//{{V2}}
DATA_BLOCK DB2000

AUTHOR:WinCoCT
FAMILY:nb
NAME:0
VERSION:00.01


       STRUCT
         VAR0:STRUCT
            VAR1:WORD
            VAR2:BYTE
            VAR3:BYTE
            VAR4:DWORD
            VAR5:BYTE
            VAR6:BYTE
            VAR7:WORD
            VAR8:BYTE
            VAR9:WORD
            VAR10:BYTE
            VAR11:WORD
            VAR12:BYTE
            VAR13:WORD
            VAR14:BYTE
            VAR15:BYTE
            VAR16:BYTE
            VAR17:BYTE
            VAR18:BYTE
            VAR19:BYTE
            VAR20:BYTE
            VAR21:BYTE
            VAR22:WORD
            VAR23:WORD
         END_STRUCT
         VAR24:STRUCT
            VAR25:WORD
            VAR26:ARRAY [0..1735] of BYTE
         END_STRUCT
         VAR27:STRUCT
            VAR28:WORD
            VAR29:ARRAY [0..79] of BYTE
         END_STRUCT
       END_STRUCT
BEGIN

       VAR0.VAR1:=W#16#0024
       VAR0.VAR2:=B#16#00
       VAR0.VAR3:=B#16#01
       VAR0.VAR4:=DW#16#00000195
       VAR0.VAR5:=B#16#01
       VAR0.VAR6:=B#16#00
       VAR0.VAR7:=W#16#0010
       VAR0.VAR8:=B#16#10
       VAR0.VAR9:=W#16#0010
       VAR0.VAR10:=B#16#10
       VAR0.VAR11:=W#16#0080
       VAR0.VAR12:=B#16#50
       VAR0.VAR13:=W#16#0080
       VAR0.VAR14:=B#16#50
       VAR0.VAR15:=B#16#02
       VAR0.VAR16:=B#16#32
       VAR0.VAR17:=B#16#01
       VAR0.VAR18:=B#16#00
       VAR0.VAR19:=B#16#01
       VAR0.VAR20:=B#16#00
       VAR0.VAR21:=B#16#00
       VAR0.VAR22:=W#16#0100
       VAR0.VAR23:=W#16#26F5
       VAR24.VAR25:=W#16#06CA
       VAR24.VAR26[0]:=B#16#4D
       VAR24.VAR26[1]:=B#16#41
       VAR24.VAR26[2]:=B#16#0A
       VAR24.VAR26[3]:=B#16#06
       VAR24.VAR26[4]:=B#16#00
       VAR24.VAR26[5]:=B#16#00
       VAR24.VAR26[6]:=B#16#FE
       VAR24.VAR26[7]:=B#16#FF
       VAR24.VAR26[8]:=B#16#A2
       VAR24.VAR26[9]:=B#16#00
       VAR24.VAR26[10]:=B#16#00
       VAR24.VAR26[11]:=B#16#00
       VAR24.VAR26[12]:=B#16#80
       VAR24.VAR26[13]:=B#16#1F
       VAR24.VAR26[14]:=B#16#00
       VAR24.VAR26[15]:=B#16#04
       VAR24.VAR26[16]:=B#16#00
       VAR24.VAR26[17]:=B#16#00
       VAR24.VAR26[18]:=B#16#00
       VAR24.VAR26[19]:=B#16#03
       VAR24.VAR26[20]:=B#16#00
       VAR24.VAR26[21]:=B#16#00
       VAR24.VAR26[22]:=B#16#00
       VAR24.VAR26[23]:=B#16#81
       VAR24.VAR26[24]:=B#16#1F
       VAR24.VAR26[25]:=B#16#04
       VAR24.VAR26[26]:=B#16#04
       VAR24.VAR26[27]:=B#16#00
       VAR24.VAR26[28]:=B#16#00
       VAR24.VAR26[29]:=B#16#00
       VAR24.VAR26[30]:=B#16#07
       VAR24.VAR26[31]:=B#16#03
       VAR24.VAR26[32]:=B#16#F4
       VAR24.VAR26[33]:=B#16#01
       VAR24.VAR26[34]:=B#16#00
       VAR24.VAR26[35]:=B#16#14
       VAR24.VAR26[36]:=B#16#01
       VAR24.VAR26[37]:=B#16#04
       VAR24.VAR26[38]:=B#16#00
       VAR24.VAR26[39]:=B#16#00
       VAR24.VAR26[40]:=B#16#00
       VAR24.VAR26[41]:=B#16#01
       VAR24.VAR26[42]:=B#16#02
       VAR24.VAR26[43]:=B#16#00
       VAR24.VAR26[44]:=B#16#80
       VAR24.VAR26[45]:=B#16#00
       VAR24.VAR26[46]:=B#16#16
       VAR24.VAR26[47]:=B#16#00
       VAR24.VAR26[48]:=B#16#01
       VAR24.VAR26[49]:=B#16#00
       VAR24.VAR26[50]:=B#16#00
       VAR24.VAR26[51]:=B#16#00
       VAR24.VAR26[52]:=B#16#00
       VAR24.VAR26[53]:=B#16#01
       VAR24.VAR26[54]:=B#16#14
       VAR24.VAR26[55]:=B#16#01
       VAR24.VAR26[56]:=B#16#04
       VAR24.VAR26[57]:=B#16#00
       VAR24.VAR26[58]:=B#16#00
       VAR24.VAR26[59]:=B#16#00
       VAR24.VAR26[60]:=B#16#01
       VAR24.VAR26[61]:=B#16#03
       VAR24.VAR26[62]:=B#16#00
       VAR24.VAR26[63]:=B#16#80
       VAR24.VAR26[64]:=B#16#01
       VAR24.VAR26[65]:=B#16#16
       VAR24.VAR26[66]:=B#16#00
       VAR24.VAR26[67]:=B#16#01
       VAR24.VAR26[68]:=B#16#00
       VAR24.VAR26[69]:=B#16#00
       VAR24.VAR26[70]:=B#16#00
       VAR24.VAR26[71]:=B#16#00
       VAR24.VAR26[72]:=B#16#02
       VAR24.VAR26[73]:=B#16#14
       VAR24.VAR26[74]:=B#16#01
       VAR24.VAR26[75]:=B#16#04
       VAR24.VAR26[76]:=B#16#00
       VAR24.VAR26[77]:=B#16#00
       VAR24.VAR26[78]:=B#16#00
       VAR24.VAR26[79]:=B#16#01
       VAR24.VAR26[80]:=B#16#04
       VAR24.VAR26[81]:=B#16#00
       VAR24.VAR26[82]:=B#16#80
       VAR24.VAR26[83]:=B#16#02
       VAR24.VAR26[84]:=B#16#16
       VAR24.VAR26[85]:=B#16#00
       VAR24.VAR26[86]:=B#16#01
       VAR24.VAR26[87]:=B#16#00
       VAR24.VAR26[88]:=B#16#00
       VAR24.VAR26[89]:=B#16#00
       VAR24.VAR26[90]:=B#16#00
       VAR24.VAR26[91]:=B#16#03
       VAR24.VAR26[92]:=B#16#14
       VAR24.VAR26[93]:=B#16#01
       VAR24.VAR26[94]:=B#16#04
       VAR24.VAR26[95]:=B#16#00
       VAR24.VAR26[96]:=B#16#00
       VAR24.VAR26[97]:=B#16#00
       VAR24.VAR26[98]:=B#16#01
       VAR24.VAR26[99]:=B#16#05
       VAR24.VAR26[100]:=B#16#00
       VAR24.VAR26[101]:=B#16#80
       VAR24.VAR26[102]:=B#16#03
       VAR24.VAR26[103]:=B#16#16
       VAR24.VAR26[104]:=B#16#00
       VAR24.VAR26[105]:=B#16#01
       VAR24.VAR26[106]:=B#16#00
       VAR24.VAR26[107]:=B#16#00
       VAR24.VAR26[108]:=B#16#00
       VAR24.VAR26[109]:=B#16#00
       VAR24.VAR26[110]:=B#16#04
       VAR24.VAR26[111]:=B#16#14
       VAR24.VAR26[112]:=B#16#01
       VAR24.VAR26[113]:=B#16#04
       VAR24.VAR26[114]:=B#16#00
       VAR24.VAR26[115]:=B#16#00
       VAR24.VAR26[116]:=B#16#00
       VAR24.VAR26[117]:=B#16#3D
       VAR24.VAR26[118]:=B#16#02
       VAR24.VAR26[119]:=B#16#00
       VAR24.VAR26[120]:=B#16#80
       VAR24.VAR26[121]:=B#16#04
       VAR24.VAR26[122]:=B#16#16
       VAR24.VAR26[123]:=B#16#00
       VAR24.VAR26[124]:=B#16#01
       VAR24.VAR26[125]:=B#16#00
       VAR24.VAR26[126]:=B#16#00
       VAR24.VAR26[127]:=B#16#00
       VAR24.VAR26[128]:=B#16#00
       VAR24.VAR26[129]:=B#16#05
       VAR24.VAR26[130]:=B#16#14
       VAR24.VAR26[131]:=B#16#01
       VAR24.VAR26[132]:=B#16#04
       VAR24.VAR26[133]:=B#16#00
       VAR24.VAR26[134]:=B#16#00
       VAR24.VAR26[135]:=B#16#00
       VAR24.VAR26[136]:=B#16#3D
       VAR24.VAR26[137]:=B#16#03
       VAR24.VAR26[138]:=B#16#00
       VAR24.VAR26[139]:=B#16#80
       VAR24.VAR26[140]:=B#16#05
       VAR24.VAR26[141]:=B#16#16
       VAR24.VAR26[142]:=B#16#00
       VAR24.VAR26[143]:=B#16#01
       VAR24.VAR26[144]:=B#16#00
       VAR24.VAR26[145]:=B#16#00
       VAR24.VAR26[146]:=B#16#00
       VAR24.VAR26[147]:=B#16#00
       VAR24.VAR26[148]:=B#16#06
       VAR24.VAR26[149]:=B#16#14
       VAR24.VAR26[150]:=B#16#01
       VAR24.VAR26[151]:=B#16#04
       VAR24.VAR26[152]:=B#16#00
       VAR24.VAR26[153]:=B#16#00
       VAR24.VAR26[154]:=B#16#00
       VAR24.VAR26[155]:=B#16#3D
       VAR24.VAR26[156]:=B#16#04
       VAR24.VAR26[157]:=B#16#00
       VAR24.VAR26[158]:=B#16#80
       VAR24.VAR26[159]:=B#16#06
       VAR24.VAR26[160]:=B#16#16
       VAR24.VAR26[161]:=B#16#00
       VAR24.VAR26[162]:=B#16#01
       VAR24.VAR26[163]:=B#16#00
       VAR24.VAR26[164]:=B#16#00
       VAR24.VAR26[165]:=B#16#00
       VAR24.VAR26[166]:=B#16#00
       VAR24.VAR26[167]:=B#16#07
       VAR24.VAR26[168]:=B#16#14
       VAR24.VAR26[169]:=B#16#01
       VAR24.VAR26[170]:=B#16#04
       VAR24.VAR26[171]:=B#16#00
       VAR24.VAR26[172]:=B#16#00
       VAR24.VAR26[173]:=B#16#00
       VAR24.VAR26[174]:=B#16#3D
       VAR24.VAR26[175]:=B#16#05
       VAR24.VAR26[176]:=B#16#00
       VAR24.VAR26[177]:=B#16#80
       VAR24.VAR26[178]:=B#16#07
       VAR24.VAR26[179]:=B#16#16
       VAR24.VAR26[180]:=B#16#00
       VAR24.VAR26[181]:=B#16#01
       VAR24.VAR26[182]:=B#16#00
       VAR24.VAR26[183]:=B#16#00
       VAR24.VAR26[184]:=B#16#00
       VAR24.VAR26[185]:=B#16#00
       VAR24.VAR26[186]:=B#16#08
       VAR24.VAR26[187]:=B#16#14
       VAR24.VAR26[188]:=B#16#01
       VAR24.VAR26[189]:=B#16#04
       VAR24.VAR26[190]:=B#16#00
       VAR24.VAR26[191]:=B#16#00
       VAR24.VAR26[192]:=B#16#00
       VAR24.VAR26[193]:=B#16#3D
       VAR24.VAR26[194]:=B#16#02
       VAR24.VAR26[195]:=B#16#00
       VAR24.VAR26[196]:=B#16#80
       VAR24.VAR26[197]:=B#16#08
       VAR24.VAR26[198]:=B#16#16
       VAR24.VAR26[199]:=B#16#00
       VAR24.VAR26[200]:=B#16#01
       VAR24.VAR26[201]:=B#16#00
       VAR24.VAR26[202]:=B#16#00
       VAR24.VAR26[203]:=B#16#00
       VAR24.VAR26[204]:=B#16#00
       VAR24.VAR26[205]:=B#16#09
       VAR24.VAR26[206]:=B#16#14
       VAR24.VAR26[207]:=B#16#01
       VAR24.VAR26[208]:=B#16#04
       VAR24.VAR26[209]:=B#16#00
       VAR24.VAR26[210]:=B#16#00
       VAR24.VAR26[211]:=B#16#00
       VAR24.VAR26[212]:=B#16#3D
       VAR24.VAR26[213]:=B#16#03
       VAR24.VAR26[214]:=B#16#00
       VAR24.VAR26[215]:=B#16#80
       VAR24.VAR26[216]:=B#16#09
       VAR24.VAR26[217]:=B#16#16
       VAR24.VAR26[218]:=B#16#00
       VAR24.VAR26[219]:=B#16#01
       VAR24.VAR26[220]:=B#16#00
       VAR24.VAR26[221]:=B#16#00
       VAR24.VAR26[222]:=B#16#00
       VAR24.VAR26[223]:=B#16#00
       VAR24.VAR26[224]:=B#16#0A
       VAR24.VAR26[225]:=B#16#14
       VAR24.VAR26[226]:=B#16#01
       VAR24.VAR26[227]:=B#16#04
       VAR24.VAR26[228]:=B#16#00
       VAR24.VAR26[229]:=B#16#00
       VAR24.VAR26[230]:=B#16#00
       VAR24.VAR26[231]:=B#16#3D
       VAR24.VAR26[232]:=B#16#04
       VAR24.VAR26[233]:=B#16#00
       VAR24.VAR26[234]:=B#16#80
       VAR24.VAR26[235]:=B#16#0A
       VAR24.VAR26[236]:=B#16#16
       VAR24.VAR26[237]:=B#16#00
       VAR24.VAR26[238]:=B#16#01
       VAR24.VAR26[239]:=B#16#00
       VAR24.VAR26[240]:=B#16#00
       VAR24.VAR26[241]:=B#16#00
       VAR24.VAR26[242]:=B#16#00
       VAR24.VAR26[243]:=B#16#0B
       VAR24.VAR26[244]:=B#16#14
       VAR24.VAR26[245]:=B#16#01
       VAR24.VAR26[246]:=B#16#04
       VAR24.VAR26[247]:=B#16#00
       VAR24.VAR26[248]:=B#16#00
       VAR24.VAR26[249]:=B#16#00
       VAR24.VAR26[250]:=B#16#3D
       VAR24.VAR26[251]:=B#16#05
       VAR24.VAR26[252]:=B#16#00
       VAR24.VAR26[253]:=B#16#80
       VAR24.VAR26[254]:=B#16#0B
       VAR24.VAR26[255]:=B#16#16
       VAR24.VAR26[256]:=B#16#00
       VAR24.VAR26[257]:=B#16#01
       VAR24.VAR26[258]:=B#16#00
       VAR24.VAR26[259]:=B#16#00
       VAR24.VAR26[260]:=B#16#00
       VAR24.VAR26[261]:=B#16#00
       VAR24.VAR26[262]:=B#16#0C
       VAR24.VAR26[263]:=B#16#14
       VAR24.VAR26[264]:=B#16#01
       VAR24.VAR26[265]:=B#16#04
       VAR24.VAR26[266]:=B#16#00
       VAR24.VAR26[267]:=B#16#00
       VAR24.VAR26[268]:=B#16#00
       VAR24.VAR26[269]:=B#16#3D
       VAR24.VAR26[270]:=B#16#02
       VAR24.VAR26[271]:=B#16#00
       VAR24.VAR26[272]:=B#16#80
       VAR24.VAR26[273]:=B#16#0C
       VAR24.VAR26[274]:=B#16#16
       VAR24.VAR26[275]:=B#16#00
       VAR24.VAR26[276]:=B#16#01
       VAR24.VAR26[277]:=B#16#00
       VAR24.VAR26[278]:=B#16#00
       VAR24.VAR26[279]:=B#16#00
       VAR24.VAR26[280]:=B#16#00
       VAR24.VAR26[281]:=B#16#0D
       VAR24.VAR26[282]:=B#16#14
       VAR24.VAR26[283]:=B#16#01
       VAR24.VAR26[284]:=B#16#04
       VAR24.VAR26[285]:=B#16#00
       VAR24.VAR26[286]:=B#16#00
       VAR24.VAR26[287]:=B#16#00
       VAR24.VAR26[288]:=B#16#3D
       VAR24.VAR26[289]:=B#16#03
       VAR24.VAR26[290]:=B#16#00
       VAR24.VAR26[291]:=B#16#80
       VAR24.VAR26[292]:=B#16#0D
       VAR24.VAR26[293]:=B#16#16
       VAR24.VAR26[294]:=B#16#00
       VAR24.VAR26[295]:=B#16#01
       VAR24.VAR26[296]:=B#16#00
       VAR24.VAR26[297]:=B#16#00
       VAR24.VAR26[298]:=B#16#00
       VAR24.VAR26[299]:=B#16#00
       VAR24.VAR26[300]:=B#16#0E
       VAR24.VAR26[301]:=B#16#14
       VAR24.VAR26[302]:=B#16#01
       VAR24.VAR26[303]:=B#16#04
       VAR24.VAR26[304]:=B#16#00
       VAR24.VAR26[305]:=B#16#00
       VAR24.VAR26[306]:=B#16#00
       VAR24.VAR26[307]:=B#16#3D
       VAR24.VAR26[308]:=B#16#04
       VAR24.VAR26[309]:=B#16#00
       VAR24.VAR26[310]:=B#16#80
       VAR24.VAR26[311]:=B#16#0E
       VAR24.VAR26[312]:=B#16#16
       VAR24.VAR26[313]:=B#16#00
       VAR24.VAR26[314]:=B#16#01
       VAR24.VAR26[315]:=B#16#00
       VAR24.VAR26[316]:=B#16#00
       VAR24.VAR26[317]:=B#16#00
       VAR24.VAR26[318]:=B#16#00
       VAR24.VAR26[319]:=B#16#0F
       VAR24.VAR26[320]:=B#16#14
       VAR24.VAR26[321]:=B#16#01
       VAR24.VAR26[322]:=B#16#04
       VAR24.VAR26[323]:=B#16#00
       VAR24.VAR26[324]:=B#16#00
       VAR24.VAR26[325]:=B#16#00
       VAR24.VAR26[326]:=B#16#3D
       VAR24.VAR26[327]:=B#16#05
       VAR24.VAR26[328]:=B#16#00
       VAR24.VAR26[329]:=B#16#80
       VAR24.VAR26[330]:=B#16#0F
       VAR24.VAR26[331]:=B#16#16
       VAR24.VAR26[332]:=B#16#00
       VAR24.VAR26[333]:=B#16#01
       VAR24.VAR26[334]:=B#16#00
       VAR24.VAR26[335]:=B#16#00
       VAR24.VAR26[336]:=B#16#00
       VAR24.VAR26[337]:=B#16#00
       VAR24.VAR26[338]:=B#16#10
       VAR24.VAR26[339]:=B#16#14
       VAR24.VAR26[340]:=B#16#01
       VAR24.VAR26[341]:=B#16#04
       VAR24.VAR26[342]:=B#16#00
       VAR24.VAR26[343]:=B#16#00
       VAR24.VAR26[344]:=B#16#00
       VAR24.VAR26[345]:=B#16#3D
       VAR24.VAR26[346]:=B#16#02
       VAR24.VAR26[347]:=B#16#00
       VAR24.VAR26[348]:=B#16#80
       VAR24.VAR26[349]:=B#16#10
       VAR24.VAR26[350]:=B#16#16
       VAR24.VAR26[351]:=B#16#00
       VAR24.VAR26[352]:=B#16#01
       VAR24.VAR26[353]:=B#16#00
       VAR24.VAR26[354]:=B#16#00
       VAR24.VAR26[355]:=B#16#00
       VAR24.VAR26[356]:=B#16#00
       VAR24.VAR26[357]:=B#16#11
       VAR24.VAR26[358]:=B#16#14
       VAR24.VAR26[359]:=B#16#01
       VAR24.VAR26[360]:=B#16#04
       VAR24.VAR26[361]:=B#16#00
       VAR24.VAR26[362]:=B#16#00
       VAR24.VAR26[363]:=B#16#00
       VAR24.VAR26[364]:=B#16#3D
       VAR24.VAR26[365]:=B#16#03
       VAR24.VAR26[366]:=B#16#00
       VAR24.VAR26[367]:=B#16#80
       VAR24.VAR26[368]:=B#16#11
       VAR24.VAR26[369]:=B#16#16
       VAR24.VAR26[370]:=B#16#00
       VAR24.VAR26[371]:=B#16#01
       VAR24.VAR26[372]:=B#16#00
       VAR24.VAR26[373]:=B#16#00
       VAR24.VAR26[374]:=B#16#00
       VAR24.VAR26[375]:=B#16#00
       VAR24.VAR26[376]:=B#16#12
       VAR24.VAR26[377]:=B#16#14
       VAR24.VAR26[378]:=B#16#01
       VAR24.VAR26[379]:=B#16#04
       VAR24.VAR26[380]:=B#16#00
       VAR24.VAR26[381]:=B#16#00
       VAR24.VAR26[382]:=B#16#00
       VAR24.VAR26[383]:=B#16#3D
       VAR24.VAR26[384]:=B#16#04
       VAR24.VAR26[385]:=B#16#00
       VAR24.VAR26[386]:=B#16#80
       VAR24.VAR26[387]:=B#16#12
       VAR24.VAR26[388]:=B#16#16
       VAR24.VAR26[389]:=B#16#00
       VAR24.VAR26[390]:=B#16#01
       VAR24.VAR26[391]:=B#16#00
       VAR24.VAR26[392]:=B#16#00
       VAR24.VAR26[393]:=B#16#00
       VAR24.VAR26[394]:=B#16#00
       VAR24.VAR26[395]:=B#16#13
       VAR24.VAR26[396]:=B#16#14
       VAR24.VAR26[397]:=B#16#01
       VAR24.VAR26[398]:=B#16#04
       VAR24.VAR26[399]:=B#16#00
       VAR24.VAR26[400]:=B#16#00
       VAR24.VAR26[401]:=B#16#00
       VAR24.VAR26[402]:=B#16#3D
       VAR24.VAR26[403]:=B#16#05
       VAR24.VAR26[404]:=B#16#00
       VAR24.VAR26[405]:=B#16#80
       VAR24.VAR26[406]:=B#16#13
       VAR24.VAR26[407]:=B#16#16
       VAR24.VAR26[408]:=B#16#00
       VAR24.VAR26[409]:=B#16#01
       VAR24.VAR26[410]:=B#16#00
       VAR24.VAR26[411]:=B#16#00
       VAR24.VAR26[412]:=B#16#00
       VAR24.VAR26[413]:=B#16#00
       VAR24.VAR26[414]:=B#16#14
       VAR24.VAR26[415]:=B#16#14
       VAR24.VAR26[416]:=B#16#01
       VAR24.VAR26[417]:=B#16#04
       VAR24.VAR26[418]:=B#16#00
       VAR24.VAR26[419]:=B#16#00
       VAR24.VAR26[420]:=B#16#00
       VAR24.VAR26[421]:=B#16#3D
       VAR24.VAR26[422]:=B#16#02
       VAR24.VAR26[423]:=B#16#00
       VAR24.VAR26[424]:=B#16#80
       VAR24.VAR26[425]:=B#16#14
       VAR24.VAR26[426]:=B#16#16
       VAR24.VAR26[427]:=B#16#00
       VAR24.VAR26[428]:=B#16#01
       VAR24.VAR26[429]:=B#16#00
       VAR24.VAR26[430]:=B#16#00
       VAR24.VAR26[431]:=B#16#00
       VAR24.VAR26[432]:=B#16#00
       VAR24.VAR26[433]:=B#16#15
       VAR24.VAR26[434]:=B#16#14
       VAR24.VAR26[435]:=B#16#01
       VAR24.VAR26[436]:=B#16#04
       VAR24.VAR26[437]:=B#16#00
       VAR24.VAR26[438]:=B#16#00
       VAR24.VAR26[439]:=B#16#00
       VAR24.VAR26[440]:=B#16#3D
       VAR24.VAR26[441]:=B#16#03
       VAR24.VAR26[442]:=B#16#00
       VAR24.VAR26[443]:=B#16#80
       VAR24.VAR26[444]:=B#16#15
       VAR24.VAR26[445]:=B#16#16
       VAR24.VAR26[446]:=B#16#00
       VAR24.VAR26[447]:=B#16#01
       VAR24.VAR26[448]:=B#16#00
       VAR24.VAR26[449]:=B#16#00
       VAR24.VAR26[450]:=B#16#00
       VAR24.VAR26[451]:=B#16#00
       VAR24.VAR26[452]:=B#16#16
       VAR24.VAR26[453]:=B#16#14
       VAR24.VAR26[454]:=B#16#01
       VAR24.VAR26[455]:=B#16#04
       VAR24.VAR26[456]:=B#16#00
       VAR24.VAR26[457]:=B#16#00
       VAR24.VAR26[458]:=B#16#00
       VAR24.VAR26[459]:=B#16#3D
       VAR24.VAR26[460]:=B#16#04
       VAR24.VAR26[461]:=B#16#00
       VAR24.VAR26[462]:=B#16#80
       VAR24.VAR26[463]:=B#16#16
       VAR24.VAR26[464]:=B#16#16
       VAR24.VAR26[465]:=B#16#00
       VAR24.VAR26[466]:=B#16#01
       VAR24.VAR26[467]:=B#16#00
       VAR24.VAR26[468]:=B#16#00
       VAR24.VAR26[469]:=B#16#00
       VAR24.VAR26[470]:=B#16#00
       VAR24.VAR26[471]:=B#16#17
       VAR24.VAR26[472]:=B#16#14
       VAR24.VAR26[473]:=B#16#01
       VAR24.VAR26[474]:=B#16#04
       VAR24.VAR26[475]:=B#16#00
       VAR24.VAR26[476]:=B#16#00
       VAR24.VAR26[477]:=B#16#00
       VAR24.VAR26[478]:=B#16#3D
       VAR24.VAR26[479]:=B#16#05
       VAR24.VAR26[480]:=B#16#00
       VAR24.VAR26[481]:=B#16#80
       VAR24.VAR26[482]:=B#16#17
       VAR24.VAR26[483]:=B#16#16
       VAR24.VAR26[484]:=B#16#00
       VAR24.VAR26[485]:=B#16#01
       VAR24.VAR26[486]:=B#16#00
       VAR24.VAR26[487]:=B#16#00
       VAR24.VAR26[488]:=B#16#00
       VAR24.VAR26[489]:=B#16#00
       VAR24.VAR26[490]:=B#16#18
       VAR24.VAR26[491]:=B#16#14
       VAR24.VAR26[492]:=B#16#01
       VAR24.VAR26[493]:=B#16#04
       VAR24.VAR26[494]:=B#16#00
       VAR24.VAR26[495]:=B#16#00
       VAR24.VAR26[496]:=B#16#00
       VAR24.VAR26[497]:=B#16#3D
       VAR24.VAR26[498]:=B#16#02
       VAR24.VAR26[499]:=B#16#00
       VAR24.VAR26[500]:=B#16#80
       VAR24.VAR26[501]:=B#16#18
       VAR24.VAR26[502]:=B#16#16
       VAR24.VAR26[503]:=B#16#00
       VAR24.VAR26[504]:=B#16#01
       VAR24.VAR26[505]:=B#16#00
       VAR24.VAR26[506]:=B#16#00
       VAR24.VAR26[507]:=B#16#00
       VAR24.VAR26[508]:=B#16#00
       VAR24.VAR26[509]:=B#16#19
       VAR24.VAR26[510]:=B#16#14
       VAR24.VAR26[511]:=B#16#01
       VAR24.VAR26[512]:=B#16#04
       VAR24.VAR26[513]:=B#16#00
       VAR24.VAR26[514]:=B#16#00
       VAR24.VAR26[515]:=B#16#00
       VAR24.VAR26[516]:=B#16#3D
       VAR24.VAR26[517]:=B#16#03
       VAR24.VAR26[518]:=B#16#00
       VAR24.VAR26[519]:=B#16#80
       VAR24.VAR26[520]:=B#16#19
       VAR24.VAR26[521]:=B#16#16
       VAR24.VAR26[522]:=B#16#00
       VAR24.VAR26[523]:=B#16#01
       VAR24.VAR26[524]:=B#16#00
       VAR24.VAR26[525]:=B#16#00
       VAR24.VAR26[526]:=B#16#00
       VAR24.VAR26[527]:=B#16#00
       VAR24.VAR26[528]:=B#16#1A
       VAR24.VAR26[529]:=B#16#14
       VAR24.VAR26[530]:=B#16#01
       VAR24.VAR26[531]:=B#16#04
       VAR24.VAR26[532]:=B#16#00
       VAR24.VAR26[533]:=B#16#00
       VAR24.VAR26[534]:=B#16#00
       VAR24.VAR26[535]:=B#16#3D
       VAR24.VAR26[536]:=B#16#04
       VAR24.VAR26[537]:=B#16#00
       VAR24.VAR26[538]:=B#16#80
       VAR24.VAR26[539]:=B#16#1A
       VAR24.VAR26[540]:=B#16#16
       VAR24.VAR26[541]:=B#16#00
       VAR24.VAR26[542]:=B#16#01
       VAR24.VAR26[543]:=B#16#00
       VAR24.VAR26[544]:=B#16#00
       VAR24.VAR26[545]:=B#16#00
       VAR24.VAR26[546]:=B#16#00
       VAR24.VAR26[547]:=B#16#1B
       VAR24.VAR26[548]:=B#16#14
       VAR24.VAR26[549]:=B#16#01
       VAR24.VAR26[550]:=B#16#04
       VAR24.VAR26[551]:=B#16#00
       VAR24.VAR26[552]:=B#16#00
       VAR24.VAR26[553]:=B#16#00
       VAR24.VAR26[554]:=B#16#3D
       VAR24.VAR26[555]:=B#16#05
       VAR24.VAR26[556]:=B#16#00
       VAR24.VAR26[557]:=B#16#80
       VAR24.VAR26[558]:=B#16#1B
       VAR24.VAR26[559]:=B#16#16
       VAR24.VAR26[560]:=B#16#00
       VAR24.VAR26[561]:=B#16#01
       VAR24.VAR26[562]:=B#16#00
       VAR24.VAR26[563]:=B#16#00
       VAR24.VAR26[564]:=B#16#00
       VAR24.VAR26[565]:=B#16#00
       VAR24.VAR26[566]:=B#16#1C
       VAR24.VAR26[567]:=B#16#14
       VAR24.VAR26[568]:=B#16#01
       VAR24.VAR26[569]:=B#16#04
       VAR24.VAR26[570]:=B#16#00
       VAR24.VAR26[571]:=B#16#00
       VAR24.VAR26[572]:=B#16#00
       VAR24.VAR26[573]:=B#16#3D
       VAR24.VAR26[574]:=B#16#02
       VAR24.VAR26[575]:=B#16#00
       VAR24.VAR26[576]:=B#16#80
       VAR24.VAR26[577]:=B#16#1C
       VAR24.VAR26[578]:=B#16#16
       VAR24.VAR26[579]:=B#16#00
       VAR24.VAR26[580]:=B#16#01
       VAR24.VAR26[581]:=B#16#00
       VAR24.VAR26[582]:=B#16#00
       VAR24.VAR26[583]:=B#16#00
       VAR24.VAR26[584]:=B#16#00
       VAR24.VAR26[585]:=B#16#1D
       VAR24.VAR26[586]:=B#16#14
       VAR24.VAR26[587]:=B#16#01
       VAR24.VAR26[588]:=B#16#04
       VAR24.VAR26[589]:=B#16#00
       VAR24.VAR26[590]:=B#16#00
       VAR24.VAR26[591]:=B#16#00
       VAR24.VAR26[592]:=B#16#3D
       VAR24.VAR26[593]:=B#16#03
       VAR24.VAR26[594]:=B#16#00
       VAR24.VAR26[595]:=B#16#80
       VAR24.VAR26[596]:=B#16#1D
       VAR24.VAR26[597]:=B#16#16
       VAR24.VAR26[598]:=B#16#00
       VAR24.VAR26[599]:=B#16#01
       VAR24.VAR26[600]:=B#16#00
       VAR24.VAR26[601]:=B#16#00
       VAR24.VAR26[602]:=B#16#00
       VAR24.VAR26[603]:=B#16#00
       VAR24.VAR26[604]:=B#16#1E
       VAR24.VAR26[605]:=B#16#14
       VAR24.VAR26[606]:=B#16#01
       VAR24.VAR26[607]:=B#16#04
       VAR24.VAR26[608]:=B#16#00
       VAR24.VAR26[609]:=B#16#00
       VAR24.VAR26[610]:=B#16#00
       VAR24.VAR26[611]:=B#16#3D
       VAR24.VAR26[612]:=B#16#04
       VAR24.VAR26[613]:=B#16#00
       VAR24.VAR26[614]:=B#16#80
       VAR24.VAR26[615]:=B#16#1E
       VAR24.VAR26[616]:=B#16#16
       VAR24.VAR26[617]:=B#16#00
       VAR24.VAR26[618]:=B#16#01
       VAR24.VAR26[619]:=B#16#00
       VAR24.VAR26[620]:=B#16#00
       VAR24.VAR26[621]:=B#16#00
       VAR24.VAR26[622]:=B#16#00
       VAR24.VAR26[623]:=B#16#1F
       VAR24.VAR26[624]:=B#16#14
       VAR24.VAR26[625]:=B#16#01
       VAR24.VAR26[626]:=B#16#04
       VAR24.VAR26[627]:=B#16#00
       VAR24.VAR26[628]:=B#16#00
       VAR24.VAR26[629]:=B#16#00
       VAR24.VAR26[630]:=B#16#3D
       VAR24.VAR26[631]:=B#16#05
       VAR24.VAR26[632]:=B#16#00
       VAR24.VAR26[633]:=B#16#80
       VAR24.VAR26[634]:=B#16#1F
       VAR24.VAR26[635]:=B#16#16
       VAR24.VAR26[636]:=B#16#00
       VAR24.VAR26[637]:=B#16#01
       VAR24.VAR26[638]:=B#16#00
       VAR24.VAR26[639]:=B#16#00
       VAR24.VAR26[640]:=B#16#00
       VAR24.VAR26[641]:=B#16#00
       VAR24.VAR26[642]:=B#16#20
       VAR24.VAR26[643]:=B#16#14
       VAR24.VAR26[644]:=B#16#01
       VAR24.VAR26[645]:=B#16#04
       VAR24.VAR26[646]:=B#16#00
       VAR24.VAR26[647]:=B#16#00
       VAR24.VAR26[648]:=B#16#00
       VAR24.VAR26[649]:=B#16#3D
       VAR24.VAR26[650]:=B#16#02
       VAR24.VAR26[651]:=B#16#00
       VAR24.VAR26[652]:=B#16#80
       VAR24.VAR26[653]:=B#16#20
       VAR24.VAR26[654]:=B#16#16
       VAR24.VAR26[655]:=B#16#00
       VAR24.VAR26[656]:=B#16#01
       VAR24.VAR26[657]:=B#16#00
       VAR24.VAR26[658]:=B#16#00
       VAR24.VAR26[659]:=B#16#00
       VAR24.VAR26[660]:=B#16#00
       VAR24.VAR26[661]:=B#16#21
       VAR24.VAR26[662]:=B#16#14
       VAR24.VAR26[663]:=B#16#01
       VAR24.VAR26[664]:=B#16#04
       VAR24.VAR26[665]:=B#16#00
       VAR24.VAR26[666]:=B#16#00
       VAR24.VAR26[667]:=B#16#00
       VAR24.VAR26[668]:=B#16#3D
       VAR24.VAR26[669]:=B#16#03
       VAR24.VAR26[670]:=B#16#00
       VAR24.VAR26[671]:=B#16#80
       VAR24.VAR26[672]:=B#16#21
       VAR24.VAR26[673]:=B#16#16
       VAR24.VAR26[674]:=B#16#00
       VAR24.VAR26[675]:=B#16#01
       VAR24.VAR26[676]:=B#16#00
       VAR24.VAR26[677]:=B#16#00
       VAR24.VAR26[678]:=B#16#00
       VAR24.VAR26[679]:=B#16#00
       VAR24.VAR26[680]:=B#16#22
       VAR24.VAR26[681]:=B#16#14
       VAR24.VAR26[682]:=B#16#01
       VAR24.VAR26[683]:=B#16#04
       VAR24.VAR26[684]:=B#16#00
       VAR24.VAR26[685]:=B#16#00
       VAR24.VAR26[686]:=B#16#00
       VAR24.VAR26[687]:=B#16#3D
       VAR24.VAR26[688]:=B#16#04
       VAR24.VAR26[689]:=B#16#00
       VAR24.VAR26[690]:=B#16#80
       VAR24.VAR26[691]:=B#16#22
       VAR24.VAR26[692]:=B#16#16
       VAR24.VAR26[693]:=B#16#00
       VAR24.VAR26[694]:=B#16#01
       VAR24.VAR26[695]:=B#16#00
       VAR24.VAR26[696]:=B#16#00
       VAR24.VAR26[697]:=B#16#00
       VAR24.VAR26[698]:=B#16#00
       VAR24.VAR26[699]:=B#16#23
       VAR24.VAR26[700]:=B#16#14
       VAR24.VAR26[701]:=B#16#01
       VAR24.VAR26[702]:=B#16#04
       VAR24.VAR26[703]:=B#16#00
       VAR24.VAR26[704]:=B#16#00
       VAR24.VAR26[705]:=B#16#00
       VAR24.VAR26[706]:=B#16#3D
       VAR24.VAR26[707]:=B#16#05
       VAR24.VAR26[708]:=B#16#00
       VAR24.VAR26[709]:=B#16#80
       VAR24.VAR26[710]:=B#16#23
       VAR24.VAR26[711]:=B#16#16
       VAR24.VAR26[712]:=B#16#00
       VAR24.VAR26[713]:=B#16#01
       VAR24.VAR26[714]:=B#16#00
       VAR24.VAR26[715]:=B#16#00
       VAR24.VAR26[716]:=B#16#00
       VAR24.VAR26[717]:=B#16#00
       VAR24.VAR26[718]:=B#16#24
       VAR24.VAR26[719]:=B#16#14
       VAR24.VAR26[720]:=B#16#01
       VAR24.VAR26[721]:=B#16#04
       VAR24.VAR26[722]:=B#16#00
       VAR24.VAR26[723]:=B#16#00
       VAR24.VAR26[724]:=B#16#00
       VAR24.VAR26[725]:=B#16#3D
       VAR24.VAR26[726]:=B#16#02
       VAR24.VAR26[727]:=B#16#00
       VAR24.VAR26[728]:=B#16#80
       VAR24.VAR26[729]:=B#16#24
       VAR24.VAR26[730]:=B#16#16
       VAR24.VAR26[731]:=B#16#00
       VAR24.VAR26[732]:=B#16#01
       VAR24.VAR26[733]:=B#16#00
       VAR24.VAR26[734]:=B#16#00
       VAR24.VAR26[735]:=B#16#00
       VAR24.VAR26[736]:=B#16#00
       VAR24.VAR26[737]:=B#16#25
       VAR24.VAR26[738]:=B#16#14
       VAR24.VAR26[739]:=B#16#01
       VAR24.VAR26[740]:=B#16#04
       VAR24.VAR26[741]:=B#16#00
       VAR24.VAR26[742]:=B#16#00
       VAR24.VAR26[743]:=B#16#00
       VAR24.VAR26[744]:=B#16#3D
       VAR24.VAR26[745]:=B#16#03
       VAR24.VAR26[746]:=B#16#00
       VAR24.VAR26[747]:=B#16#80
       VAR24.VAR26[748]:=B#16#25
       VAR24.VAR26[749]:=B#16#16
       VAR24.VAR26[750]:=B#16#00
       VAR24.VAR26[751]:=B#16#01
       VAR24.VAR26[752]:=B#16#00
       VAR24.VAR26[753]:=B#16#00
       VAR24.VAR26[754]:=B#16#00
       VAR24.VAR26[755]:=B#16#00
       VAR24.VAR26[756]:=B#16#26
       VAR24.VAR26[757]:=B#16#14
       VAR24.VAR26[758]:=B#16#01
       VAR24.VAR26[759]:=B#16#04
       VAR24.VAR26[760]:=B#16#00
       VAR24.VAR26[761]:=B#16#00
       VAR24.VAR26[762]:=B#16#00
       VAR24.VAR26[763]:=B#16#3D
       VAR24.VAR26[764]:=B#16#04
       VAR24.VAR26[765]:=B#16#00
       VAR24.VAR26[766]:=B#16#80
       VAR24.VAR26[767]:=B#16#26
       VAR24.VAR26[768]:=B#16#16
       VAR24.VAR26[769]:=B#16#00
       VAR24.VAR26[770]:=B#16#01
       VAR24.VAR26[771]:=B#16#00
       VAR24.VAR26[772]:=B#16#00
       VAR24.VAR26[773]:=B#16#00
       VAR24.VAR26[774]:=B#16#00
       VAR24.VAR26[775]:=B#16#27
       VAR24.VAR26[776]:=B#16#14
       VAR24.VAR26[777]:=B#16#01
       VAR24.VAR26[778]:=B#16#04
       VAR24.VAR26[779]:=B#16#00
       VAR24.VAR26[780]:=B#16#00
       VAR24.VAR26[781]:=B#16#00
       VAR24.VAR26[782]:=B#16#3D
       VAR24.VAR26[783]:=B#16#05
       VAR24.VAR26[784]:=B#16#00
       VAR24.VAR26[785]:=B#16#80
       VAR24.VAR26[786]:=B#16#27
       VAR24.VAR26[787]:=B#16#16
       VAR24.VAR26[788]:=B#16#00
       VAR24.VAR26[789]:=B#16#01
       VAR24.VAR26[790]:=B#16#00
       VAR24.VAR26[791]:=B#16#00
       VAR24.VAR26[792]:=B#16#00
       VAR24.VAR26[793]:=B#16#00
       VAR24.VAR26[794]:=B#16#00
       VAR24.VAR26[795]:=B#16#18
       VAR24.VAR26[796]:=B#16#01
       VAR24.VAR26[797]:=B#16#04
       VAR24.VAR26[798]:=B#16#00
       VAR24.VAR26[799]:=B#16#00
       VAR24.VAR26[800]:=B#16#00
       VAR24.VAR26[801]:=B#16#81
       VAR24.VAR26[802]:=B#16#01
       VAR24.VAR26[803]:=B#16#00
       VAR24.VAR26[804]:=B#16#80
       VAR24.VAR26[805]:=B#16#00
       VAR24.VAR26[806]:=B#16#1A
       VAR24.VAR26[807]:=B#16#00
       VAR24.VAR26[808]:=B#16#01
       VAR24.VAR26[809]:=B#16#00
       VAR24.VAR26[810]:=B#16#00
       VAR24.VAR26[811]:=B#16#00
       VAR24.VAR26[812]:=B#16#00
       VAR24.VAR26[813]:=B#16#01
       VAR24.VAR26[814]:=B#16#18
       VAR24.VAR26[815]:=B#16#01
       VAR24.VAR26[816]:=B#16#04
       VAR24.VAR26[817]:=B#16#00
       VAR24.VAR26[818]:=B#16#00
       VAR24.VAR26[819]:=B#16#00
       VAR24.VAR26[820]:=B#16#81
       VAR24.VAR26[821]:=B#16#02
       VAR24.VAR26[822]:=B#16#00
       VAR24.VAR26[823]:=B#16#80
       VAR24.VAR26[824]:=B#16#01
       VAR24.VAR26[825]:=B#16#1A
       VAR24.VAR26[826]:=B#16#00
       VAR24.VAR26[827]:=B#16#01
       VAR24.VAR26[828]:=B#16#00
       VAR24.VAR26[829]:=B#16#00
       VAR24.VAR26[830]:=B#16#00
       VAR24.VAR26[831]:=B#16#00
       VAR24.VAR26[832]:=B#16#02
       VAR24.VAR26[833]:=B#16#18
       VAR24.VAR26[834]:=B#16#01
       VAR24.VAR26[835]:=B#16#04
       VAR24.VAR26[836]:=B#16#00
       VAR24.VAR26[837]:=B#16#00
       VAR24.VAR26[838]:=B#16#00
       VAR24.VAR26[839]:=B#16#81
       VAR24.VAR26[840]:=B#16#03
       VAR24.VAR26[841]:=B#16#00
       VAR24.VAR26[842]:=B#16#80
       VAR24.VAR26[843]:=B#16#02
       VAR24.VAR26[844]:=B#16#1A
       VAR24.VAR26[845]:=B#16#00
       VAR24.VAR26[846]:=B#16#01
       VAR24.VAR26[847]:=B#16#00
       VAR24.VAR26[848]:=B#16#00
       VAR24.VAR26[849]:=B#16#00
       VAR24.VAR26[850]:=B#16#00
       VAR24.VAR26[851]:=B#16#03
       VAR24.VAR26[852]:=B#16#18
       VAR24.VAR26[853]:=B#16#01
       VAR24.VAR26[854]:=B#16#04
       VAR24.VAR26[855]:=B#16#00
       VAR24.VAR26[856]:=B#16#00
       VAR24.VAR26[857]:=B#16#00
       VAR24.VAR26[858]:=B#16#81
       VAR24.VAR26[859]:=B#16#04
       VAR24.VAR26[860]:=B#16#00
       VAR24.VAR26[861]:=B#16#80
       VAR24.VAR26[862]:=B#16#03
       VAR24.VAR26[863]:=B#16#1A
       VAR24.VAR26[864]:=B#16#00
       VAR24.VAR26[865]:=B#16#01
       VAR24.VAR26[866]:=B#16#00
       VAR24.VAR26[867]:=B#16#00
       VAR24.VAR26[868]:=B#16#00
       VAR24.VAR26[869]:=B#16#00
       VAR24.VAR26[870]:=B#16#04
       VAR24.VAR26[871]:=B#16#18
       VAR24.VAR26[872]:=B#16#01
       VAR24.VAR26[873]:=B#16#04
       VAR24.VAR26[874]:=B#16#00
       VAR24.VAR26[875]:=B#16#00
       VAR24.VAR26[876]:=B#16#00
       VAR24.VAR26[877]:=B#16#BD
       VAR24.VAR26[878]:=B#16#01
       VAR24.VAR26[879]:=B#16#00
       VAR24.VAR26[880]:=B#16#80
       VAR24.VAR26[881]:=B#16#04
       VAR24.VAR26[882]:=B#16#1A
       VAR24.VAR26[883]:=B#16#00
       VAR24.VAR26[884]:=B#16#01
       VAR24.VAR26[885]:=B#16#00
       VAR24.VAR26[886]:=B#16#00
       VAR24.VAR26[887]:=B#16#00
       VAR24.VAR26[888]:=B#16#00
       VAR24.VAR26[889]:=B#16#05
       VAR24.VAR26[890]:=B#16#18
       VAR24.VAR26[891]:=B#16#01
       VAR24.VAR26[892]:=B#16#04
       VAR24.VAR26[893]:=B#16#00
       VAR24.VAR26[894]:=B#16#00
       VAR24.VAR26[895]:=B#16#00
       VAR24.VAR26[896]:=B#16#BD
       VAR24.VAR26[897]:=B#16#02
       VAR24.VAR26[898]:=B#16#00
       VAR24.VAR26[899]:=B#16#80
       VAR24.VAR26[900]:=B#16#05
       VAR24.VAR26[901]:=B#16#1A
       VAR24.VAR26[902]:=B#16#00
       VAR24.VAR26[903]:=B#16#01
       VAR24.VAR26[904]:=B#16#00
       VAR24.VAR26[905]:=B#16#00
       VAR24.VAR26[906]:=B#16#00
       VAR24.VAR26[907]:=B#16#00
       VAR24.VAR26[908]:=B#16#06
       VAR24.VAR26[909]:=B#16#18
       VAR24.VAR26[910]:=B#16#01
       VAR24.VAR26[911]:=B#16#04
       VAR24.VAR26[912]:=B#16#00
       VAR24.VAR26[913]:=B#16#00
       VAR24.VAR26[914]:=B#16#00
       VAR24.VAR26[915]:=B#16#BD
       VAR24.VAR26[916]:=B#16#03
       VAR24.VAR26[917]:=B#16#00
       VAR24.VAR26[918]:=B#16#80
       VAR24.VAR26[919]:=B#16#06
       VAR24.VAR26[920]:=B#16#1A
       VAR24.VAR26[921]:=B#16#00
       VAR24.VAR26[922]:=B#16#01
       VAR24.VAR26[923]:=B#16#00
       VAR24.VAR26[924]:=B#16#00
       VAR24.VAR26[925]:=B#16#00
       VAR24.VAR26[926]:=B#16#00
       VAR24.VAR26[927]:=B#16#07
       VAR24.VAR26[928]:=B#16#18
       VAR24.VAR26[929]:=B#16#01
       VAR24.VAR26[930]:=B#16#04
       VAR24.VAR26[931]:=B#16#00
       VAR24.VAR26[932]:=B#16#00
       VAR24.VAR26[933]:=B#16#00
       VAR24.VAR26[934]:=B#16#BD
       VAR24.VAR26[935]:=B#16#04
       VAR24.VAR26[936]:=B#16#00
       VAR24.VAR26[937]:=B#16#80
       VAR24.VAR26[938]:=B#16#07
       VAR24.VAR26[939]:=B#16#1A
       VAR24.VAR26[940]:=B#16#00
       VAR24.VAR26[941]:=B#16#01
       VAR24.VAR26[942]:=B#16#00
       VAR24.VAR26[943]:=B#16#00
       VAR24.VAR26[944]:=B#16#00
       VAR24.VAR26[945]:=B#16#00
       VAR24.VAR26[946]:=B#16#08
       VAR24.VAR26[947]:=B#16#18
       VAR24.VAR26[948]:=B#16#01
       VAR24.VAR26[949]:=B#16#04
       VAR24.VAR26[950]:=B#16#00
       VAR24.VAR26[951]:=B#16#00
       VAR24.VAR26[952]:=B#16#00
       VAR24.VAR26[953]:=B#16#BD
       VAR24.VAR26[954]:=B#16#01
       VAR24.VAR26[955]:=B#16#00
       VAR24.VAR26[956]:=B#16#80
       VAR24.VAR26[957]:=B#16#08
       VAR24.VAR26[958]:=B#16#1A
       VAR24.VAR26[959]:=B#16#00
       VAR24.VAR26[960]:=B#16#01
       VAR24.VAR26[961]:=B#16#00
       VAR24.VAR26[962]:=B#16#00
       VAR24.VAR26[963]:=B#16#00
       VAR24.VAR26[964]:=B#16#00
       VAR24.VAR26[965]:=B#16#09
       VAR24.VAR26[966]:=B#16#18
       VAR24.VAR26[967]:=B#16#01
       VAR24.VAR26[968]:=B#16#04
       VAR24.VAR26[969]:=B#16#00
       VAR24.VAR26[970]:=B#16#00
       VAR24.VAR26[971]:=B#16#00
       VAR24.VAR26[972]:=B#16#BD
       VAR24.VAR26[973]:=B#16#02
       VAR24.VAR26[974]:=B#16#00
       VAR24.VAR26[975]:=B#16#80
       VAR24.VAR26[976]:=B#16#09
       VAR24.VAR26[977]:=B#16#1A
       VAR24.VAR26[978]:=B#16#00
       VAR24.VAR26[979]:=B#16#01
       VAR24.VAR26[980]:=B#16#00
       VAR24.VAR26[981]:=B#16#00
       VAR24.VAR26[982]:=B#16#00
       VAR24.VAR26[983]:=B#16#00
       VAR24.VAR26[984]:=B#16#0A
       VAR24.VAR26[985]:=B#16#18
       VAR24.VAR26[986]:=B#16#01
       VAR24.VAR26[987]:=B#16#04
       VAR24.VAR26[988]:=B#16#00
       VAR24.VAR26[989]:=B#16#00
       VAR24.VAR26[990]:=B#16#00
       VAR24.VAR26[991]:=B#16#BD
       VAR24.VAR26[992]:=B#16#03
       VAR24.VAR26[993]:=B#16#00
       VAR24.VAR26[994]:=B#16#80
       VAR24.VAR26[995]:=B#16#0A
       VAR24.VAR26[996]:=B#16#1A
       VAR24.VAR26[997]:=B#16#00
       VAR24.VAR26[998]:=B#16#01
       VAR24.VAR26[999]:=B#16#00
       VAR24.VAR26[1000]:=B#16#00
       VAR24.VAR26[1001]:=B#16#00
       VAR24.VAR26[1002]:=B#16#00
       VAR24.VAR26[1003]:=B#16#0B
       VAR24.VAR26[1004]:=B#16#18
       VAR24.VAR26[1005]:=B#16#01
       VAR24.VAR26[1006]:=B#16#04
       VAR24.VAR26[1007]:=B#16#00
       VAR24.VAR26[1008]:=B#16#00
       VAR24.VAR26[1009]:=B#16#00
       VAR24.VAR26[1010]:=B#16#BD
       VAR24.VAR26[1011]:=B#16#04
       VAR24.VAR26[1012]:=B#16#00
       VAR24.VAR26[1013]:=B#16#80
       VAR24.VAR26[1014]:=B#16#0B
       VAR24.VAR26[1015]:=B#16#1A
       VAR24.VAR26[1016]:=B#16#00
       VAR24.VAR26[1017]:=B#16#01
       VAR24.VAR26[1018]:=B#16#00
       VAR24.VAR26[1019]:=B#16#00
       VAR24.VAR26[1020]:=B#16#00
       VAR24.VAR26[1021]:=B#16#00
       VAR24.VAR26[1022]:=B#16#0C
       VAR24.VAR26[1023]:=B#16#18
       VAR24.VAR26[1024]:=B#16#01
       VAR24.VAR26[1025]:=B#16#04
       VAR24.VAR26[1026]:=B#16#00
       VAR24.VAR26[1027]:=B#16#00
       VAR24.VAR26[1028]:=B#16#00
       VAR24.VAR26[1029]:=B#16#BD
       VAR24.VAR26[1030]:=B#16#01
       VAR24.VAR26[1031]:=B#16#00
       VAR24.VAR26[1032]:=B#16#80
       VAR24.VAR26[1033]:=B#16#0C
       VAR24.VAR26[1034]:=B#16#1A
       VAR24.VAR26[1035]:=B#16#00
       VAR24.VAR26[1036]:=B#16#01
       VAR24.VAR26[1037]:=B#16#00
       VAR24.VAR26[1038]:=B#16#00
       VAR24.VAR26[1039]:=B#16#00
       VAR24.VAR26[1040]:=B#16#00
       VAR24.VAR26[1041]:=B#16#0D
       VAR24.VAR26[1042]:=B#16#18
       VAR24.VAR26[1043]:=B#16#01
       VAR24.VAR26[1044]:=B#16#04
       VAR24.VAR26[1045]:=B#16#00
       VAR24.VAR26[1046]:=B#16#00
       VAR24.VAR26[1047]:=B#16#00
       VAR24.VAR26[1048]:=B#16#BD
       VAR24.VAR26[1049]:=B#16#02
       VAR24.VAR26[1050]:=B#16#00
       VAR24.VAR26[1051]:=B#16#80
       VAR24.VAR26[1052]:=B#16#0D
       VAR24.VAR26[1053]:=B#16#1A
       VAR24.VAR26[1054]:=B#16#00
       VAR24.VAR26[1055]:=B#16#01
       VAR24.VAR26[1056]:=B#16#00
       VAR24.VAR26[1057]:=B#16#00
       VAR24.VAR26[1058]:=B#16#00
       VAR24.VAR26[1059]:=B#16#00
       VAR24.VAR26[1060]:=B#16#0E
       VAR24.VAR26[1061]:=B#16#18
       VAR24.VAR26[1062]:=B#16#01
       VAR24.VAR26[1063]:=B#16#04
       VAR24.VAR26[1064]:=B#16#00
       VAR24.VAR26[1065]:=B#16#00
       VAR24.VAR26[1066]:=B#16#00
       VAR24.VAR26[1067]:=B#16#BD
       VAR24.VAR26[1068]:=B#16#03
       VAR24.VAR26[1069]:=B#16#00
       VAR24.VAR26[1070]:=B#16#80
       VAR24.VAR26[1071]:=B#16#0E
       VAR24.VAR26[1072]:=B#16#1A
       VAR24.VAR26[1073]:=B#16#00
       VAR24.VAR26[1074]:=B#16#01
       VAR24.VAR26[1075]:=B#16#00
       VAR24.VAR26[1076]:=B#16#00
       VAR24.VAR26[1077]:=B#16#00
       VAR24.VAR26[1078]:=B#16#00
       VAR24.VAR26[1079]:=B#16#0F
       VAR24.VAR26[1080]:=B#16#18
       VAR24.VAR26[1081]:=B#16#01
       VAR24.VAR26[1082]:=B#16#04
       VAR24.VAR26[1083]:=B#16#00
       VAR24.VAR26[1084]:=B#16#00
       VAR24.VAR26[1085]:=B#16#00
       VAR24.VAR26[1086]:=B#16#BD
       VAR24.VAR26[1087]:=B#16#04
       VAR24.VAR26[1088]:=B#16#00
       VAR24.VAR26[1089]:=B#16#80
       VAR24.VAR26[1090]:=B#16#0F
       VAR24.VAR26[1091]:=B#16#1A
       VAR24.VAR26[1092]:=B#16#00
       VAR24.VAR26[1093]:=B#16#01
       VAR24.VAR26[1094]:=B#16#00
       VAR24.VAR26[1095]:=B#16#00
       VAR24.VAR26[1096]:=B#16#00
       VAR24.VAR26[1097]:=B#16#00
       VAR24.VAR26[1098]:=B#16#10
       VAR24.VAR26[1099]:=B#16#18
       VAR24.VAR26[1100]:=B#16#01
       VAR24.VAR26[1101]:=B#16#04
       VAR24.VAR26[1102]:=B#16#00
       VAR24.VAR26[1103]:=B#16#00
       VAR24.VAR26[1104]:=B#16#00
       VAR24.VAR26[1105]:=B#16#BD
       VAR24.VAR26[1106]:=B#16#01
       VAR24.VAR26[1107]:=B#16#00
       VAR24.VAR26[1108]:=B#16#80
       VAR24.VAR26[1109]:=B#16#10
       VAR24.VAR26[1110]:=B#16#1A
       VAR24.VAR26[1111]:=B#16#00
       VAR24.VAR26[1112]:=B#16#01
       VAR24.VAR26[1113]:=B#16#00
       VAR24.VAR26[1114]:=B#16#00
       VAR24.VAR26[1115]:=B#16#00
       VAR24.VAR26[1116]:=B#16#00
       VAR24.VAR26[1117]:=B#16#11
       VAR24.VAR26[1118]:=B#16#18
       VAR24.VAR26[1119]:=B#16#01
       VAR24.VAR26[1120]:=B#16#04
       VAR24.VAR26[1121]:=B#16#00
       VAR24.VAR26[1122]:=B#16#00
       VAR24.VAR26[1123]:=B#16#00
       VAR24.VAR26[1124]:=B#16#BD
       VAR24.VAR26[1125]:=B#16#02
       VAR24.VAR26[1126]:=B#16#00
       VAR24.VAR26[1127]:=B#16#80
       VAR24.VAR26[1128]:=B#16#11
       VAR24.VAR26[1129]:=B#16#1A
       VAR24.VAR26[1130]:=B#16#00
       VAR24.VAR26[1131]:=B#16#01
       VAR24.VAR26[1132]:=B#16#00
       VAR24.VAR26[1133]:=B#16#00
       VAR24.VAR26[1134]:=B#16#00
       VAR24.VAR26[1135]:=B#16#00
       VAR24.VAR26[1136]:=B#16#12
       VAR24.VAR26[1137]:=B#16#18
       VAR24.VAR26[1138]:=B#16#01
       VAR24.VAR26[1139]:=B#16#04
       VAR24.VAR26[1140]:=B#16#00
       VAR24.VAR26[1141]:=B#16#00
       VAR24.VAR26[1142]:=B#16#00
       VAR24.VAR26[1143]:=B#16#BD
       VAR24.VAR26[1144]:=B#16#03
       VAR24.VAR26[1145]:=B#16#00
       VAR24.VAR26[1146]:=B#16#80
       VAR24.VAR26[1147]:=B#16#12
       VAR24.VAR26[1148]:=B#16#1A
       VAR24.VAR26[1149]:=B#16#00
       VAR24.VAR26[1150]:=B#16#01
       VAR24.VAR26[1151]:=B#16#00
       VAR24.VAR26[1152]:=B#16#00
       VAR24.VAR26[1153]:=B#16#00
       VAR24.VAR26[1154]:=B#16#00
       VAR24.VAR26[1155]:=B#16#13
       VAR24.VAR26[1156]:=B#16#18
       VAR24.VAR26[1157]:=B#16#01
       VAR24.VAR26[1158]:=B#16#04
       VAR24.VAR26[1159]:=B#16#00
       VAR24.VAR26[1160]:=B#16#00
       VAR24.VAR26[1161]:=B#16#00
       VAR24.VAR26[1162]:=B#16#BD
       VAR24.VAR26[1163]:=B#16#04
       VAR24.VAR26[1164]:=B#16#00
       VAR24.VAR26[1165]:=B#16#80
       VAR24.VAR26[1166]:=B#16#13
       VAR24.VAR26[1167]:=B#16#1A
       VAR24.VAR26[1168]:=B#16#00
       VAR24.VAR26[1169]:=B#16#01
       VAR24.VAR26[1170]:=B#16#00
       VAR24.VAR26[1171]:=B#16#00
       VAR24.VAR26[1172]:=B#16#00
       VAR24.VAR26[1173]:=B#16#00
       VAR24.VAR26[1174]:=B#16#14
       VAR24.VAR26[1175]:=B#16#18
       VAR24.VAR26[1176]:=B#16#01
       VAR24.VAR26[1177]:=B#16#04
       VAR24.VAR26[1178]:=B#16#00
       VAR24.VAR26[1179]:=B#16#00
       VAR24.VAR26[1180]:=B#16#00
       VAR24.VAR26[1181]:=B#16#BD
       VAR24.VAR26[1182]:=B#16#01
       VAR24.VAR26[1183]:=B#16#00
       VAR24.VAR26[1184]:=B#16#80
       VAR24.VAR26[1185]:=B#16#14
       VAR24.VAR26[1186]:=B#16#1A
       VAR24.VAR26[1187]:=B#16#00
       VAR24.VAR26[1188]:=B#16#01
       VAR24.VAR26[1189]:=B#16#00
       VAR24.VAR26[1190]:=B#16#00
       VAR24.VAR26[1191]:=B#16#00
       VAR24.VAR26[1192]:=B#16#00
       VAR24.VAR26[1193]:=B#16#15
       VAR24.VAR26[1194]:=B#16#18
       VAR24.VAR26[1195]:=B#16#01
       VAR24.VAR26[1196]:=B#16#04
       VAR24.VAR26[1197]:=B#16#00
       VAR24.VAR26[1198]:=B#16#00
       VAR24.VAR26[1199]:=B#16#00
       VAR24.VAR26[1200]:=B#16#BD
       VAR24.VAR26[1201]:=B#16#02
       VAR24.VAR26[1202]:=B#16#00
       VAR24.VAR26[1203]:=B#16#80
       VAR24.VAR26[1204]:=B#16#15
       VAR24.VAR26[1205]:=B#16#1A
       VAR24.VAR26[1206]:=B#16#00
       VAR24.VAR26[1207]:=B#16#01
       VAR24.VAR26[1208]:=B#16#00
       VAR24.VAR26[1209]:=B#16#00
       VAR24.VAR26[1210]:=B#16#00
       VAR24.VAR26[1211]:=B#16#00
       VAR24.VAR26[1212]:=B#16#16
       VAR24.VAR26[1213]:=B#16#18
       VAR24.VAR26[1214]:=B#16#01
       VAR24.VAR26[1215]:=B#16#04
       VAR24.VAR26[1216]:=B#16#00
       VAR24.VAR26[1217]:=B#16#00
       VAR24.VAR26[1218]:=B#16#00
       VAR24.VAR26[1219]:=B#16#BD
       VAR24.VAR26[1220]:=B#16#03
       VAR24.VAR26[1221]:=B#16#00
       VAR24.VAR26[1222]:=B#16#80
       VAR24.VAR26[1223]:=B#16#16
       VAR24.VAR26[1224]:=B#16#1A
       VAR24.VAR26[1225]:=B#16#00
       VAR24.VAR26[1226]:=B#16#01
       VAR24.VAR26[1227]:=B#16#00
       VAR24.VAR26[1228]:=B#16#00
       VAR24.VAR26[1229]:=B#16#00
       VAR24.VAR26[1230]:=B#16#00
       VAR24.VAR26[1231]:=B#16#17
       VAR24.VAR26[1232]:=B#16#18
       VAR24.VAR26[1233]:=B#16#01
       VAR24.VAR26[1234]:=B#16#04
       VAR24.VAR26[1235]:=B#16#00
       VAR24.VAR26[1236]:=B#16#00
       VAR24.VAR26[1237]:=B#16#00
       VAR24.VAR26[1238]:=B#16#BD
       VAR24.VAR26[1239]:=B#16#04
       VAR24.VAR26[1240]:=B#16#00
       VAR24.VAR26[1241]:=B#16#80
       VAR24.VAR26[1242]:=B#16#17
       VAR24.VAR26[1243]:=B#16#1A
       VAR24.VAR26[1244]:=B#16#00
       VAR24.VAR26[1245]:=B#16#01
       VAR24.VAR26[1246]:=B#16#00
       VAR24.VAR26[1247]:=B#16#00
       VAR24.VAR26[1248]:=B#16#00
       VAR24.VAR26[1249]:=B#16#00
       VAR24.VAR26[1250]:=B#16#18
       VAR24.VAR26[1251]:=B#16#18
       VAR24.VAR26[1252]:=B#16#01
       VAR24.VAR26[1253]:=B#16#04
       VAR24.VAR26[1254]:=B#16#00
       VAR24.VAR26[1255]:=B#16#00
       VAR24.VAR26[1256]:=B#16#00
       VAR24.VAR26[1257]:=B#16#BD
       VAR24.VAR26[1258]:=B#16#01
       VAR24.VAR26[1259]:=B#16#00
       VAR24.VAR26[1260]:=B#16#80
       VAR24.VAR26[1261]:=B#16#18
       VAR24.VAR26[1262]:=B#16#1A
       VAR24.VAR26[1263]:=B#16#00
       VAR24.VAR26[1264]:=B#16#01
       VAR24.VAR26[1265]:=B#16#00
       VAR24.VAR26[1266]:=B#16#00
       VAR24.VAR26[1267]:=B#16#00
       VAR24.VAR26[1268]:=B#16#00
       VAR24.VAR26[1269]:=B#16#19
       VAR24.VAR26[1270]:=B#16#18
       VAR24.VAR26[1271]:=B#16#01
       VAR24.VAR26[1272]:=B#16#04
       VAR24.VAR26[1273]:=B#16#00
       VAR24.VAR26[1274]:=B#16#00
       VAR24.VAR26[1275]:=B#16#00
       VAR24.VAR26[1276]:=B#16#BD
       VAR24.VAR26[1277]:=B#16#02
       VAR24.VAR26[1278]:=B#16#00
       VAR24.VAR26[1279]:=B#16#80
       VAR24.VAR26[1280]:=B#16#19
       VAR24.VAR26[1281]:=B#16#1A
       VAR24.VAR26[1282]:=B#16#00
       VAR24.VAR26[1283]:=B#16#01
       VAR24.VAR26[1284]:=B#16#00
       VAR24.VAR26[1285]:=B#16#00
       VAR24.VAR26[1286]:=B#16#00
       VAR24.VAR26[1287]:=B#16#00
       VAR24.VAR26[1288]:=B#16#1A
       VAR24.VAR26[1289]:=B#16#18
       VAR24.VAR26[1290]:=B#16#01
       VAR24.VAR26[1291]:=B#16#04
       VAR24.VAR26[1292]:=B#16#00
       VAR24.VAR26[1293]:=B#16#00
       VAR24.VAR26[1294]:=B#16#00
       VAR24.VAR26[1295]:=B#16#BD
       VAR24.VAR26[1296]:=B#16#03
       VAR24.VAR26[1297]:=B#16#00
       VAR24.VAR26[1298]:=B#16#80
       VAR24.VAR26[1299]:=B#16#1A
       VAR24.VAR26[1300]:=B#16#1A
       VAR24.VAR26[1301]:=B#16#00
       VAR24.VAR26[1302]:=B#16#01
       VAR24.VAR26[1303]:=B#16#00
       VAR24.VAR26[1304]:=B#16#00
       VAR24.VAR26[1305]:=B#16#00
       VAR24.VAR26[1306]:=B#16#00
       VAR24.VAR26[1307]:=B#16#1B
       VAR24.VAR26[1308]:=B#16#18
       VAR24.VAR26[1309]:=B#16#01
       VAR24.VAR26[1310]:=B#16#04
       VAR24.VAR26[1311]:=B#16#00
       VAR24.VAR26[1312]:=B#16#00
       VAR24.VAR26[1313]:=B#16#00
       VAR24.VAR26[1314]:=B#16#BD
       VAR24.VAR26[1315]:=B#16#04
       VAR24.VAR26[1316]:=B#16#00
       VAR24.VAR26[1317]:=B#16#80
       VAR24.VAR26[1318]:=B#16#1B
       VAR24.VAR26[1319]:=B#16#1A
       VAR24.VAR26[1320]:=B#16#00
       VAR24.VAR26[1321]:=B#16#01
       VAR24.VAR26[1322]:=B#16#00
       VAR24.VAR26[1323]:=B#16#00
       VAR24.VAR26[1324]:=B#16#00
       VAR24.VAR26[1325]:=B#16#00
       VAR24.VAR26[1326]:=B#16#1C
       VAR24.VAR26[1327]:=B#16#18
       VAR24.VAR26[1328]:=B#16#01
       VAR24.VAR26[1329]:=B#16#04
       VAR24.VAR26[1330]:=B#16#00
       VAR24.VAR26[1331]:=B#16#00
       VAR24.VAR26[1332]:=B#16#00
       VAR24.VAR26[1333]:=B#16#BD
       VAR24.VAR26[1334]:=B#16#01
       VAR24.VAR26[1335]:=B#16#00
       VAR24.VAR26[1336]:=B#16#80
       VAR24.VAR26[1337]:=B#16#1C
       VAR24.VAR26[1338]:=B#16#1A
       VAR24.VAR26[1339]:=B#16#00
       VAR24.VAR26[1340]:=B#16#01
       VAR24.VAR26[1341]:=B#16#00
       VAR24.VAR26[1342]:=B#16#00
       VAR24.VAR26[1343]:=B#16#00
       VAR24.VAR26[1344]:=B#16#00
       VAR24.VAR26[1345]:=B#16#1D
       VAR24.VAR26[1346]:=B#16#18
       VAR24.VAR26[1347]:=B#16#01
       VAR24.VAR26[1348]:=B#16#04
       VAR24.VAR26[1349]:=B#16#00
       VAR24.VAR26[1350]:=B#16#00
       VAR24.VAR26[1351]:=B#16#00
       VAR24.VAR26[1352]:=B#16#BD
       VAR24.VAR26[1353]:=B#16#02
       VAR24.VAR26[1354]:=B#16#00
       VAR24.VAR26[1355]:=B#16#80
       VAR24.VAR26[1356]:=B#16#1D
       VAR24.VAR26[1357]:=B#16#1A
       VAR24.VAR26[1358]:=B#16#00
       VAR24.VAR26[1359]:=B#16#01
       VAR24.VAR26[1360]:=B#16#00
       VAR24.VAR26[1361]:=B#16#00
       VAR24.VAR26[1362]:=B#16#00
       VAR24.VAR26[1363]:=B#16#00
       VAR24.VAR26[1364]:=B#16#1E
       VAR24.VAR26[1365]:=B#16#18
       VAR24.VAR26[1366]:=B#16#01
       VAR24.VAR26[1367]:=B#16#04
       VAR24.VAR26[1368]:=B#16#00
       VAR24.VAR26[1369]:=B#16#00
       VAR24.VAR26[1370]:=B#16#00
       VAR24.VAR26[1371]:=B#16#BD
       VAR24.VAR26[1372]:=B#16#03
       VAR24.VAR26[1373]:=B#16#00
       VAR24.VAR26[1374]:=B#16#80
       VAR24.VAR26[1375]:=B#16#1E
       VAR24.VAR26[1376]:=B#16#1A
       VAR24.VAR26[1377]:=B#16#00
       VAR24.VAR26[1378]:=B#16#01
       VAR24.VAR26[1379]:=B#16#00
       VAR24.VAR26[1380]:=B#16#00
       VAR24.VAR26[1381]:=B#16#00
       VAR24.VAR26[1382]:=B#16#00
       VAR24.VAR26[1383]:=B#16#1F
       VAR24.VAR26[1384]:=B#16#18
       VAR24.VAR26[1385]:=B#16#01
       VAR24.VAR26[1386]:=B#16#04
       VAR24.VAR26[1387]:=B#16#00
       VAR24.VAR26[1388]:=B#16#00
       VAR24.VAR26[1389]:=B#16#00
       VAR24.VAR26[1390]:=B#16#BD
       VAR24.VAR26[1391]:=B#16#04
       VAR24.VAR26[1392]:=B#16#00
       VAR24.VAR26[1393]:=B#16#80
       VAR24.VAR26[1394]:=B#16#1F
       VAR24.VAR26[1395]:=B#16#1A
       VAR24.VAR26[1396]:=B#16#00
       VAR24.VAR26[1397]:=B#16#01
       VAR24.VAR26[1398]:=B#16#00
       VAR24.VAR26[1399]:=B#16#00
       VAR24.VAR26[1400]:=B#16#00
       VAR24.VAR26[1401]:=B#16#00
       VAR24.VAR26[1402]:=B#16#20
       VAR24.VAR26[1403]:=B#16#18
       VAR24.VAR26[1404]:=B#16#01
       VAR24.VAR26[1405]:=B#16#04
       VAR24.VAR26[1406]:=B#16#00
       VAR24.VAR26[1407]:=B#16#00
       VAR24.VAR26[1408]:=B#16#00
       VAR24.VAR26[1409]:=B#16#BD
       VAR24.VAR26[1410]:=B#16#01
       VAR24.VAR26[1411]:=B#16#00
       VAR24.VAR26[1412]:=B#16#80
       VAR24.VAR26[1413]:=B#16#20
       VAR24.VAR26[1414]:=B#16#1A
       VAR24.VAR26[1415]:=B#16#00
       VAR24.VAR26[1416]:=B#16#01
       VAR24.VAR26[1417]:=B#16#00
       VAR24.VAR26[1418]:=B#16#00
       VAR24.VAR26[1419]:=B#16#00
       VAR24.VAR26[1420]:=B#16#00
       VAR24.VAR26[1421]:=B#16#21
       VAR24.VAR26[1422]:=B#16#18
       VAR24.VAR26[1423]:=B#16#01
       VAR24.VAR26[1424]:=B#16#04
       VAR24.VAR26[1425]:=B#16#00
       VAR24.VAR26[1426]:=B#16#00
       VAR24.VAR26[1427]:=B#16#00
       VAR24.VAR26[1428]:=B#16#BD
       VAR24.VAR26[1429]:=B#16#02
       VAR24.VAR26[1430]:=B#16#00
       VAR24.VAR26[1431]:=B#16#80
       VAR24.VAR26[1432]:=B#16#21
       VAR24.VAR26[1433]:=B#16#1A
       VAR24.VAR26[1434]:=B#16#00
       VAR24.VAR26[1435]:=B#16#01
       VAR24.VAR26[1436]:=B#16#00
       VAR24.VAR26[1437]:=B#16#00
       VAR24.VAR26[1438]:=B#16#00
       VAR24.VAR26[1439]:=B#16#00
       VAR24.VAR26[1440]:=B#16#22
       VAR24.VAR26[1441]:=B#16#18
       VAR24.VAR26[1442]:=B#16#01
       VAR24.VAR26[1443]:=B#16#04
       VAR24.VAR26[1444]:=B#16#00
       VAR24.VAR26[1445]:=B#16#00
       VAR24.VAR26[1446]:=B#16#00
       VAR24.VAR26[1447]:=B#16#BD
       VAR24.VAR26[1448]:=B#16#03
       VAR24.VAR26[1449]:=B#16#00
       VAR24.VAR26[1450]:=B#16#80
       VAR24.VAR26[1451]:=B#16#22
       VAR24.VAR26[1452]:=B#16#1A
       VAR24.VAR26[1453]:=B#16#00
       VAR24.VAR26[1454]:=B#16#01
       VAR24.VAR26[1455]:=B#16#00
       VAR24.VAR26[1456]:=B#16#00
       VAR24.VAR26[1457]:=B#16#00
       VAR24.VAR26[1458]:=B#16#00
       VAR24.VAR26[1459]:=B#16#23
       VAR24.VAR26[1460]:=B#16#18
       VAR24.VAR26[1461]:=B#16#01
       VAR24.VAR26[1462]:=B#16#04
       VAR24.VAR26[1463]:=B#16#00
       VAR24.VAR26[1464]:=B#16#00
       VAR24.VAR26[1465]:=B#16#00
       VAR24.VAR26[1466]:=B#16#BD
       VAR24.VAR26[1467]:=B#16#04
       VAR24.VAR26[1468]:=B#16#00
       VAR24.VAR26[1469]:=B#16#80
       VAR24.VAR26[1470]:=B#16#23
       VAR24.VAR26[1471]:=B#16#1A
       VAR24.VAR26[1472]:=B#16#00
       VAR24.VAR26[1473]:=B#16#01
       VAR24.VAR26[1474]:=B#16#00
       VAR24.VAR26[1475]:=B#16#00
       VAR24.VAR26[1476]:=B#16#00
       VAR24.VAR26[1477]:=B#16#00
       VAR24.VAR26[1478]:=B#16#24
       VAR24.VAR26[1479]:=B#16#18
       VAR24.VAR26[1480]:=B#16#01
       VAR24.VAR26[1481]:=B#16#04
       VAR24.VAR26[1482]:=B#16#00
       VAR24.VAR26[1483]:=B#16#00
       VAR24.VAR26[1484]:=B#16#00
       VAR24.VAR26[1485]:=B#16#BD
       VAR24.VAR26[1486]:=B#16#01
       VAR24.VAR26[1487]:=B#16#00
       VAR24.VAR26[1488]:=B#16#80
       VAR24.VAR26[1489]:=B#16#24
       VAR24.VAR26[1490]:=B#16#1A
       VAR24.VAR26[1491]:=B#16#00
       VAR24.VAR26[1492]:=B#16#01
       VAR24.VAR26[1493]:=B#16#00
       VAR24.VAR26[1494]:=B#16#00
       VAR24.VAR26[1495]:=B#16#00
       VAR24.VAR26[1496]:=B#16#00
       VAR24.VAR26[1497]:=B#16#25
       VAR24.VAR26[1498]:=B#16#18
       VAR24.VAR26[1499]:=B#16#01
       VAR24.VAR26[1500]:=B#16#04
       VAR24.VAR26[1501]:=B#16#00
       VAR24.VAR26[1502]:=B#16#00
       VAR24.VAR26[1503]:=B#16#00
       VAR24.VAR26[1504]:=B#16#BD
       VAR24.VAR26[1505]:=B#16#02
       VAR24.VAR26[1506]:=B#16#00
       VAR24.VAR26[1507]:=B#16#80
       VAR24.VAR26[1508]:=B#16#25
       VAR24.VAR26[1509]:=B#16#1A
       VAR24.VAR26[1510]:=B#16#00
       VAR24.VAR26[1511]:=B#16#01
       VAR24.VAR26[1512]:=B#16#00
       VAR24.VAR26[1513]:=B#16#00
       VAR24.VAR26[1514]:=B#16#00
       VAR24.VAR26[1515]:=B#16#00
       VAR24.VAR26[1516]:=B#16#26
       VAR24.VAR26[1517]:=B#16#18
       VAR24.VAR26[1518]:=B#16#01
       VAR24.VAR26[1519]:=B#16#04
       VAR24.VAR26[1520]:=B#16#00
       VAR24.VAR26[1521]:=B#16#00
       VAR24.VAR26[1522]:=B#16#00
       VAR24.VAR26[1523]:=B#16#BD
       VAR24.VAR26[1524]:=B#16#03
       VAR24.VAR26[1525]:=B#16#00
       VAR24.VAR26[1526]:=B#16#80
       VAR24.VAR26[1527]:=B#16#26
       VAR24.VAR26[1528]:=B#16#1A
       VAR24.VAR26[1529]:=B#16#00
       VAR24.VAR26[1530]:=B#16#01
       VAR24.VAR26[1531]:=B#16#00
       VAR24.VAR26[1532]:=B#16#00
       VAR24.VAR26[1533]:=B#16#00
       VAR24.VAR26[1534]:=B#16#00
       VAR24.VAR26[1535]:=B#16#27
       VAR24.VAR26[1536]:=B#16#18
       VAR24.VAR26[1537]:=B#16#01
       VAR24.VAR26[1538]:=B#16#04
       VAR24.VAR26[1539]:=B#16#00
       VAR24.VAR26[1540]:=B#16#00
       VAR24.VAR26[1541]:=B#16#00
       VAR24.VAR26[1542]:=B#16#BD
       VAR24.VAR26[1543]:=B#16#04
       VAR24.VAR26[1544]:=B#16#00
       VAR24.VAR26[1545]:=B#16#80
       VAR24.VAR26[1546]:=B#16#27
       VAR24.VAR26[1547]:=B#16#1A
       VAR24.VAR26[1548]:=B#16#00
       VAR24.VAR26[1549]:=B#16#01
       VAR24.VAR26[1550]:=B#16#00
       VAR24.VAR26[1551]:=B#16#00
       VAR24.VAR26[1552]:=B#16#00
       VAR24.VAR26[1553]:=B#16#00
       VAR24.VAR26[1554]:=B#16#4D
       VAR24.VAR26[1555]:=B#16#41
       VAR24.VAR26[1556]:=B#16#AD
       VAR24.VAR26[1557]:=B#16#00
       VAR24.VAR26[1558]:=B#16#00
       VAR24.VAR26[1559]:=B#16#00
       VAR24.VAR26[1560]:=B#16#04
       VAR24.VAR26[1561]:=B#16#FF
       VAR24.VAR26[1562]:=B#16#12
       VAR24.VAR26[1563]:=B#16#00
       VAR24.VAR26[1564]:=B#16#00
       VAR24.VAR26[1565]:=B#16#00
       VAR24.VAR26[1566]:=B#16#0C
       VAR24.VAR26[1567]:=B#16#10
       VAR24.VAR26[1568]:=B#16#00
       VAR24.VAR26[1569]:=B#16#02
       VAR24.VAR26[1570]:=B#16#00
       VAR24.VAR26[1571]:=B#16#00
       VAR24.VAR26[1572]:=B#16#00
       VAR24.VAR26[1573]:=B#16#F4
       VAR24.VAR26[1574]:=B#16#01
       VAR24.VAR26[1575]:=B#16#0D
       VAR24.VAR26[1576]:=B#16#10
       VAR24.VAR26[1577]:=B#16#00
       VAR24.VAR26[1578]:=B#16#01
       VAR24.VAR26[1579]:=B#16#00
       VAR24.VAR26[1580]:=B#16#00
       VAR24.VAR26[1581]:=B#16#00
       VAR24.VAR26[1582]:=B#16#03
       VAR24.VAR26[1583]:=B#16#00
       VAR24.VAR26[1584]:=B#16#14
       VAR24.VAR26[1585]:=B#16#01
       VAR24.VAR26[1586]:=B#16#04
       VAR24.VAR26[1587]:=B#16#00
       VAR24.VAR26[1588]:=B#16#00
       VAR24.VAR26[1589]:=B#16#00
       VAR24.VAR26[1590]:=B#16#04
       VAR24.VAR26[1591]:=B#16#02
       VAR24.VAR26[1592]:=B#16#00
       VAR24.VAR26[1593]:=B#16#80
       VAR24.VAR26[1594]:=B#16#00
       VAR24.VAR26[1595]:=B#16#16
       VAR24.VAR26[1596]:=B#16#00
       VAR24.VAR26[1597]:=B#16#01
       VAR24.VAR26[1598]:=B#16#00
       VAR24.VAR26[1599]:=B#16#00
       VAR24.VAR26[1600]:=B#16#00
       VAR24.VAR26[1601]:=B#16#01
       VAR24.VAR26[1602]:=B#16#01
       VAR24.VAR26[1603]:=B#16#14
       VAR24.VAR26[1604]:=B#16#01
       VAR24.VAR26[1605]:=B#16#04
       VAR24.VAR26[1606]:=B#16#00
       VAR24.VAR26[1607]:=B#16#00
       VAR24.VAR26[1608]:=B#16#00
       VAR24.VAR26[1609]:=B#16#04
       VAR24.VAR26[1610]:=B#16#03
       VAR24.VAR26[1611]:=B#16#00
       VAR24.VAR26[1612]:=B#16#80
       VAR24.VAR26[1613]:=B#16#01
       VAR24.VAR26[1614]:=B#16#16
       VAR24.VAR26[1615]:=B#16#00
       VAR24.VAR26[1616]:=B#16#01
       VAR24.VAR26[1617]:=B#16#00
       VAR24.VAR26[1618]:=B#16#00
       VAR24.VAR26[1619]:=B#16#00
       VAR24.VAR26[1620]:=B#16#02
       VAR24.VAR26[1621]:=B#16#02
       VAR24.VAR26[1622]:=B#16#14
       VAR24.VAR26[1623]:=B#16#01
       VAR24.VAR26[1624]:=B#16#04
       VAR24.VAR26[1625]:=B#16#00
       VAR24.VAR26[1626]:=B#16#00
       VAR24.VAR26[1627]:=B#16#00
       VAR24.VAR26[1628]:=B#16#04
       VAR24.VAR26[1629]:=B#16#04
       VAR24.VAR26[1630]:=B#16#00
       VAR24.VAR26[1631]:=B#16#80
       VAR24.VAR26[1632]:=B#16#02
       VAR24.VAR26[1633]:=B#16#16
       VAR24.VAR26[1634]:=B#16#00
       VAR24.VAR26[1635]:=B#16#01
       VAR24.VAR26[1636]:=B#16#00
       VAR24.VAR26[1637]:=B#16#00
       VAR24.VAR26[1638]:=B#16#00
       VAR24.VAR26[1639]:=B#16#02
       VAR24.VAR26[1640]:=B#16#03
       VAR24.VAR26[1641]:=B#16#14
       VAR24.VAR26[1642]:=B#16#01
       VAR24.VAR26[1643]:=B#16#04
       VAR24.VAR26[1644]:=B#16#00
       VAR24.VAR26[1645]:=B#16#00
       VAR24.VAR26[1646]:=B#16#00
       VAR24.VAR26[1647]:=B#16#04
       VAR24.VAR26[1648]:=B#16#05
       VAR24.VAR26[1649]:=B#16#00
       VAR24.VAR26[1650]:=B#16#80
       VAR24.VAR26[1651]:=B#16#03
       VAR24.VAR26[1652]:=B#16#16
       VAR24.VAR26[1653]:=B#16#00
       VAR24.VAR26[1654]:=B#16#01
       VAR24.VAR26[1655]:=B#16#00
       VAR24.VAR26[1656]:=B#16#00
       VAR24.VAR26[1657]:=B#16#00
       VAR24.VAR26[1658]:=B#16#02
       VAR24.VAR26[1659]:=B#16#00
       VAR24.VAR26[1660]:=B#16#18
       VAR24.VAR26[1661]:=B#16#01
       VAR24.VAR26[1662]:=B#16#04
       VAR24.VAR26[1663]:=B#16#00
       VAR24.VAR26[1664]:=B#16#00
       VAR24.VAR26[1665]:=B#16#00
       VAR24.VAR26[1666]:=B#16#84
       VAR24.VAR26[1667]:=B#16#01
       VAR24.VAR26[1668]:=B#16#00
       VAR24.VAR26[1669]:=B#16#C0
       VAR24.VAR26[1670]:=B#16#00
       VAR24.VAR26[1671]:=B#16#1A
       VAR24.VAR26[1672]:=B#16#00
       VAR24.VAR26[1673]:=B#16#01
       VAR24.VAR26[1674]:=B#16#00
       VAR24.VAR26[1675]:=B#16#00
       VAR24.VAR26[1676]:=B#16#00
       VAR24.VAR26[1677]:=B#16#01
       VAR24.VAR26[1678]:=B#16#01
       VAR24.VAR26[1679]:=B#16#18
       VAR24.VAR26[1680]:=B#16#01
       VAR24.VAR26[1681]:=B#16#04
       VAR24.VAR26[1682]:=B#16#00
       VAR24.VAR26[1683]:=B#16#00
       VAR24.VAR26[1684]:=B#16#00
       VAR24.VAR26[1685]:=B#16#84
       VAR24.VAR26[1686]:=B#16#02
       VAR24.VAR26[1687]:=B#16#00
       VAR24.VAR26[1688]:=B#16#C0
       VAR24.VAR26[1689]:=B#16#01
       VAR24.VAR26[1690]:=B#16#1A
       VAR24.VAR26[1691]:=B#16#00
       VAR24.VAR26[1692]:=B#16#01
       VAR24.VAR26[1693]:=B#16#00
       VAR24.VAR26[1694]:=B#16#00
       VAR24.VAR26[1695]:=B#16#00
       VAR24.VAR26[1696]:=B#16#02
       VAR24.VAR26[1697]:=B#16#02
       VAR24.VAR26[1698]:=B#16#18
       VAR24.VAR26[1699]:=B#16#01
       VAR24.VAR26[1700]:=B#16#04
       VAR24.VAR26[1701]:=B#16#00
       VAR24.VAR26[1702]:=B#16#00
       VAR24.VAR26[1703]:=B#16#00
       VAR24.VAR26[1704]:=B#16#84
       VAR24.VAR26[1705]:=B#16#03
       VAR24.VAR26[1706]:=B#16#00
       VAR24.VAR26[1707]:=B#16#C0
       VAR24.VAR26[1708]:=B#16#02
       VAR24.VAR26[1709]:=B#16#1A
       VAR24.VAR26[1710]:=B#16#00
       VAR24.VAR26[1711]:=B#16#01
       VAR24.VAR26[1712]:=B#16#00
       VAR24.VAR26[1713]:=B#16#00
       VAR24.VAR26[1714]:=B#16#00
       VAR24.VAR26[1715]:=B#16#02
       VAR24.VAR26[1716]:=B#16#03
       VAR24.VAR26[1717]:=B#16#18
       VAR24.VAR26[1718]:=B#16#01
       VAR24.VAR26[1719]:=B#16#04
       VAR24.VAR26[1720]:=B#16#00
       VAR24.VAR26[1721]:=B#16#00
       VAR24.VAR26[1722]:=B#16#00
       VAR24.VAR26[1723]:=B#16#84
       VAR24.VAR26[1724]:=B#16#04
       VAR24.VAR26[1725]:=B#16#00
       VAR24.VAR26[1726]:=B#16#C0
       VAR24.VAR26[1727]:=B#16#03
       VAR24.VAR26[1728]:=B#16#1A
       VAR24.VAR26[1729]:=B#16#00
       VAR24.VAR26[1730]:=B#16#01
       VAR24.VAR26[1731]:=B#16#00
       VAR24.VAR26[1732]:=B#16#00
       VAR24.VAR26[1733]:=B#16#00
       VAR24.VAR26[1734]:=B#16#02
       VAR24.VAR26[1735]:=B#16#00
       VAR27.VAR28:=W#16#0052
       VAR27.VAR29[0]:=B#16#00
       VAR27.VAR29[1]:=B#16#00
       VAR27.VAR29[2]:=B#16#00
       VAR27.VAR29[3]:=B#16#00
       VAR27.VAR29[4]:=B#16#00
       VAR27.VAR29[5]:=B#16#00
       VAR27.VAR29[6]:=B#16#00
       VAR27.VAR29[7]:=B#16#00
       VAR27.VAR29[8]:=B#16#00
       VAR27.VAR29[9]:=B#16#00
       VAR27.VAR29[10]:=B#16#00
       VAR27.VAR29[11]:=B#16#00
       VAR27.VAR29[12]:=B#16#00
       VAR27.VAR29[13]:=B#16#00
       VAR27.VAR29[14]:=B#16#00
       VAR27.VAR29[15]:=B#16#00
       VAR27.VAR29[16]:=B#16#00
       VAR27.VAR29[17]:=B#16#00
       VAR27.VAR29[18]:=B#16#00
       VAR27.VAR29[19]:=B#16#00
       VAR27.VAR29[20]:=B#16#00
       VAR27.VAR29[21]:=B#16#00
       VAR27.VAR29[22]:=B#16#00
       VAR27.VAR29[23]:=B#16#00
       VAR27.VAR29[24]:=B#16#00
       VAR27.VAR29[25]:=B#16#00
       VAR27.VAR29[26]:=B#16#00
       VAR27.VAR29[27]:=B#16#00
       VAR27.VAR29[28]:=B#16#00
       VAR27.VAR29[29]:=B#16#00
       VAR27.VAR29[30]:=B#16#00
       VAR27.VAR29[31]:=B#16#00
       VAR27.VAR29[32]:=B#16#00
       VAR27.VAR29[33]:=B#16#00
       VAR27.VAR29[34]:=B#16#00
       VAR27.VAR29[35]:=B#16#00
       VAR27.VAR29[36]:=B#16#00
       VAR27.VAR29[37]:=B#16#00
       VAR27.VAR29[38]:=B#16#00
       VAR27.VAR29[39]:=B#16#00
       VAR27.VAR29[40]:=B#16#00
       VAR27.VAR29[41]:=B#16#00
       VAR27.VAR29[42]:=B#16#00
       VAR27.VAR29[43]:=B#16#00
       VAR27.VAR29[44]:=B#16#00
       VAR27.VAR29[45]:=B#16#00
       VAR27.VAR29[46]:=B#16#00
       VAR27.VAR29[47]:=B#16#00
       VAR27.VAR29[48]:=B#16#00
       VAR27.VAR29[49]:=B#16#00
       VAR27.VAR29[50]:=B#16#00
       VAR27.VAR29[51]:=B#16#00
       VAR27.VAR29[52]:=B#16#00
       VAR27.VAR29[53]:=B#16#00
       VAR27.VAR29[54]:=B#16#00
       VAR27.VAR29[55]:=B#16#00
       VAR27.VAR29[56]:=B#16#00
       VAR27.VAR29[57]:=B#16#00
       VAR27.VAR29[58]:=B#16#00
       VAR27.VAR29[59]:=B#16#00
       VAR27.VAR29[60]:=B#16#00
       VAR27.VAR29[61]:=B#16#00
       VAR27.VAR29[62]:=B#16#00
       VAR27.VAR29[63]:=B#16#00
       VAR27.VAR29[64]:=B#16#00
       VAR27.VAR29[65]:=B#16#00
       VAR27.VAR29[66]:=B#16#00
       VAR27.VAR29[67]:=B#16#00
       VAR27.VAR29[68]:=B#16#00
       VAR27.VAR29[69]:=B#16#00
       VAR27.VAR29[70]:=B#16#00
       VAR27.VAR29[71]:=B#16#00
       VAR27.VAR29[72]:=B#16#00
       VAR27.VAR29[73]:=B#16#00
       VAR27.VAR29[74]:=B#16#00
       VAR27.VAR29[75]:=B#16#00
       VAR27.VAR29[76]:=B#16#00
       VAR27.VAR29[77]:=B#16#00
       VAR27.VAR29[78]:=B#16#00
       VAR27.VAR29[79]:=B#16#00
END_DATA_BLOCK
